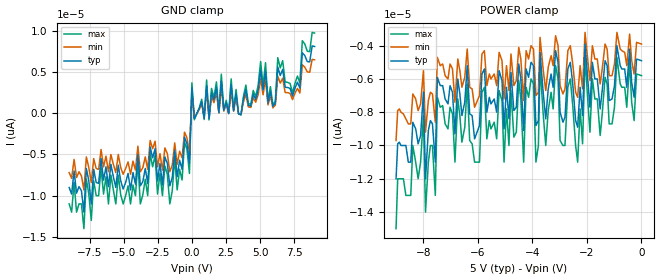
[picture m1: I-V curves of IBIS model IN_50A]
| TEXAS INSTRUMENTS INCORPORATED
| Standard Linear and Logic Group / High Volume Linear
| IBIS Model of TPD1E10B09-Q1
| Single Channel ESD Protection Device
| This file contains package information for the following:
|  QFN 2-pin (DPY) package as [Component] TPD1E10B09-Q1_DPY
| This device can be powered at the following Vccs:
|  9 volt Vcc
| This file provides unique models under the [Model Selector] for each Vcc.
| For operation at a specific Vcc, select the appropriate model after each
| [Model Selector] keyword.
[IBIS Ver]   3.2
[Comment char]  |_char
[File Name]   tpd1e10b09-q1.ibs
[File Rev]   0 | A1
[Date]   ????????
[Source]   Data created from TI-SPICE simulations at TI-SLL/HVL.
   The following is an IBIS list for the TPD1E10B09-Q1.
   Please contact sllibis@ti.com with questions and
   comments concerning SLL IBIS models.
[Notes]   Revision_History:
[Disclaimer]
| This model is designed as an aid for customers of Texas Instruments.
| TI and its licensors and suppliers make no warranties, either expressed
| or implied, with respect to this  model, including the warranties of
| merchantability or fitness for a particular purpose. The model is
| provided solely on an "as is" basis. The entire risk as to its quality
| and performance is with the customer.
[Copyright]
| (C) Copyright 2016 Texas Instruments Incorporated. All rights reserved.
| Component TPD1E10B09-Q1_DPY 2-PIN QFN
[Component]   TPD1E10B09-Q1_DPY
[Manufacturer]   Texas Instruments, Inc.
[Package]
|   typ   min   max
R_pkg   6.000e-02   5.900e-02   6.100e-02
L_pkg   5.003e-10   4.430e-10   5.015e-10
C_pkg   2.000e-14   1.990e-14   2.010e-14
[Pin]   signal_name   model_name   R_pin   L_pin   C_pin
1   1   IN_50A   6.100e-02   4.430e-10   1.990e-14
2   2   GND   6.100e-02   4.430e-10   1.990e-14
| Models and submodels in the file (1): IN_50A (Input)
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| Model IN
[Model]   IN_50A
Model_type  Input
Vinl=0
Vinh=9
| variable   typ   min   max
C_comp   9.9pF   8.9pF   10.9pF
[Temperature Range]   40   100   -40
| Ambient temperature   25   85   -40
[Voltage range]   5   5   5
[GND Clamp]
| IN_50A
|   Voltage   I(typ)   I(min)   I(max)
-9V       -9pA       -7.2pA     -11pA
-3.96V    -5pA       -4pA       -6pA
-3.78V    -8.8pA     -7.1pA     -11pA
-3.06V    -4.1pA     -3.3pA     -4.9pA
-1.62V    -8.8pA     -7.1pA     -11pA
-180mV    -6.1pA     -4.9pA     -7.3pA
0V        3.08pA     2.47pA     3.7pA
3.6V      -170fA     -140fA     -210fA
5.4V      5.12pA     4.09pA     6.14pA
5.94V     822fA      657fA      986fA
6.3V      5.61pA     4.49pA     6.74pA
9V        8.1pA      6.48pA     9.72pA
[POWER Clamp]
| IN_50A
|   Voltage   I(typ)   I(min)   I(max)
-9V       -12pA      -9.7pA     -15pA
-7.995V   -6.8pA     -5.5pA     -8.2pA
-7.92V    -12pA      -9.2pA     -14pA
-7.56V    -11pA      -8.6pA     -13pA
-7.485V   -5.9pA     -4.7pA     -7.1pA
-4.32V    -9.1pA     -7.3pA     -11pA
-4.05V    -5pA       -4pA       -6pA
-3.87V    -8.8pA     -7pA       -11pA
-3.15V    -4.3pA     -3.4pA     -5.2pA
-2.34V    -8.9pA     -7.1pA     -11pA
-2.07V    -3.9pA     -3.2pA     -4.7pA
0V        -4.9pA     -3.9pA     -5.8pA
